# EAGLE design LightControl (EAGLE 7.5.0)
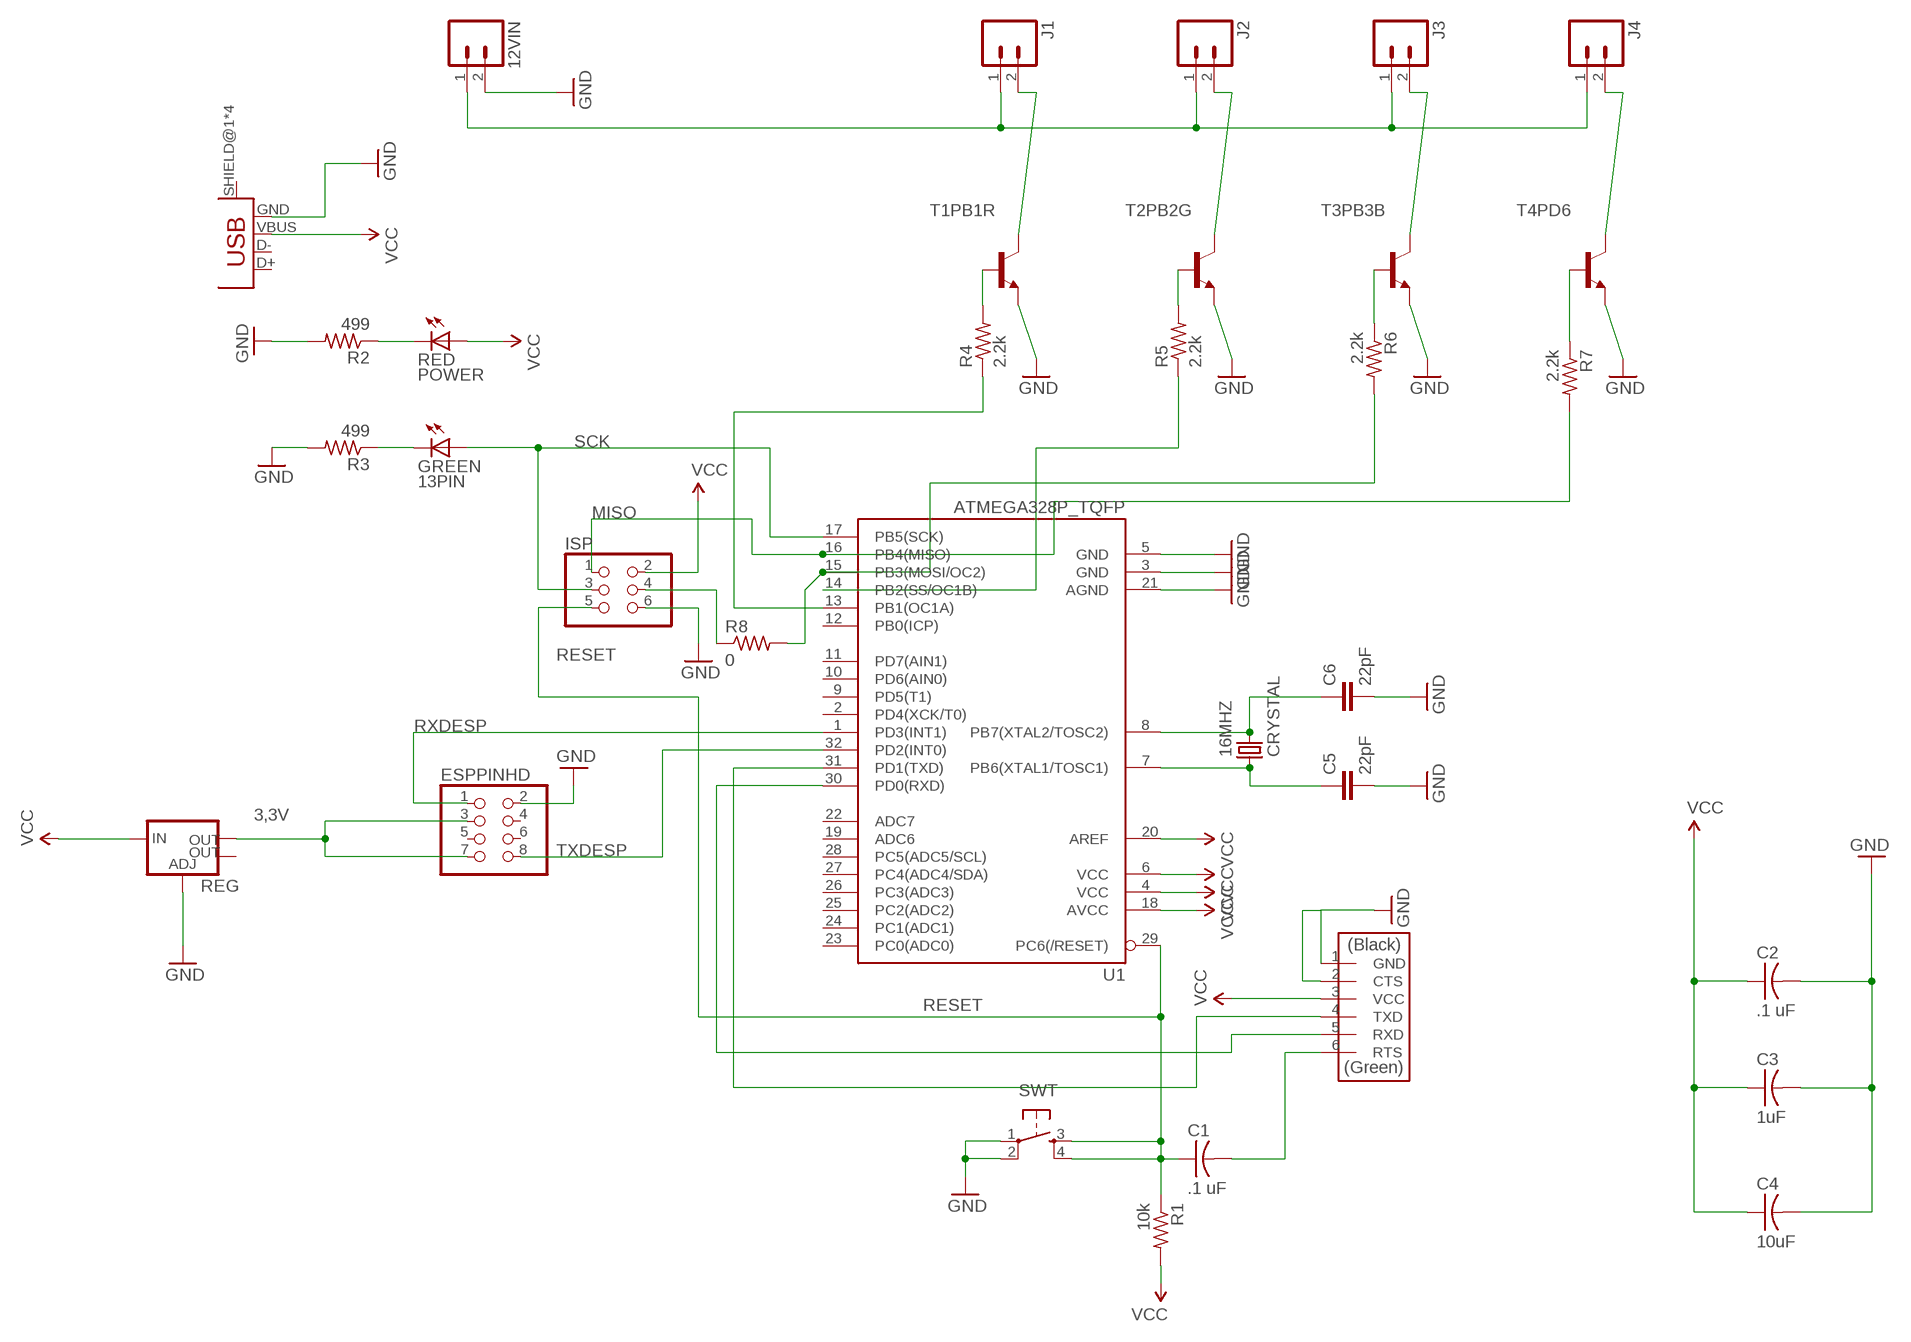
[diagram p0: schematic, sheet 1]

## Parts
12VIN  M025MM  [SCREWTERMINAL-5MM-2]
16MHZ  CRYSTAL  [2-SMD-5X3MM]
C1  .1 uF  CAP-US1206  [C1206]
C2  .1 uF  CAP-US1206  [C1206]
C3  1uF  CAP-US1206  [C1206]
C4  10uF  CAP-US1206  [C1206]
C5  22pF  CAPPTH1  [CAP-PTH-5MM]
C6  22pF  CAPPTH1  [CAP-PTH-5MM]
ESPPINHD  PINHD-2X4SMT  [2X04_SMT]
GREEN  13PIN  LEDFAB1206  [LED1206FAB]
ISP  PINHD-2X3-SMD  [2X03SMD]
J1  M025MM  [SCREWTERMINAL-5MM-2]
J2  M025MM  [SCREWTERMINAL-5MM-2]
J3  M025MM  [SCREWTERMINAL-5MM-2]
J4  M025MM  [SCREWTERMINAL-5MM-2]
R1  10k  RES-US1206FAB  [R1206FAB]
R2  499  RES-US1206FAB  [R1206FAB]
R3  499  RES-US1206FAB  [R1206FAB]
R4  2.2k  RES-US1206FAB  [R1206FAB]
R5  2.2k  RES-US1206FAB  [R1206FAB]
R6  2.2k  RES-US1206FAB  [R1206FAB]
R7  2.2k  RES-US1206FAB  [R1206FAB]
R8  0  RES-US1206FAB  [R1206FAB]
RED  POWER  LEDFAB1206  [LED1206FAB]
REG  V_REG_LM1117SOT223  [SOT223]
SWT  6MM_SWITCH6MM_SWITCH  [6MM_SWITCH]
T1PB1R  -NPN-TO220V  [TO220V]
T2PB2G  -NPN-TO220V  [TO220V]
T3PB3B  -NPN-TO220V  [TO220V]
T4PD6  -NPN-TO220V  [TO220V]
U1  ATMEGA328P_TQFP  [TQFP32-08]
U$1  FTDI-SMD-HEADER  [1X06SMD]
U$2  USB_MINIB  [USB_MINIB]

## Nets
3,3V: ESPPINHD.3 ESPPINHD.7 REG.2(OUT)
GND: 12VIN.2 C2.2 C3.2 C4.2 C5.2 C6.2 ESPPINHD.2 ISP.6 R2.2 R3.2 REG.1(ADJ) SWT.1(P) SWT.2(P1) T1PB1R.3(E) T2PB2G.3(E) T3PB3B.3(E) T4PD6.3(E) U1.3(GND) U1.5(GND) U1.21(AGND) U$1.1(GND) U$1.2(CTS) U$2.GND
MISO: ISP.1 R7.2 U1.16(PB4(MISO))
MOSI: R6.2 R8.2 U1.15(PB3(MOSI/OC2))
N$1: U1.30(PD0(RXD)) U$1.5(RXD)
N$2: 16MHZ.P$2 C6.1 U1.8(PB7(XTAL2/TOSC2))
N$3: 16MHZ.P$1 C5.1 U1.7(PB6(XTAL1/TOSC1))
N$4: C1.2 U$1.6(RTS)
N$5: R2.1 RED.2(C)
N$6: U1.31(PD1(TXD)) U$1.4(TXD)
N$7: ISP.4 R8.1
N$8: GREEN.2(C) R3.1
N$9: R4.2 T1PB1R.1(B)
N$10: R5.2 T2PB2G.1(B)
N$11: R6.1 T3PB3B.1(B)
N$12: R7.1 T4PD6.1(B)
N$13: R4.1 U1.13(PB1(OC1A))
N$14: R5.1 U1.14(PB2(SS/OC1B))
N$15: J1.2 T1PB1R.2(C)
N$16: J2.2 T2PB2G.2(C)
N$17: J3.2 T3PB3B.2(C)
N$18: J4.2 T4PD6.2(C)
N$19: 12VIN.1 J1.1 J2.1 J3.1 J4.1
RESET: C1.1 ISP.5 R1.1 SWT.3(S) SWT.4(S1) U1.29(PC6(/RESET))
RXDESP: ESPPINHD.1 U1.1(PD3(INT1))
SCK: GREEN.1(A) ISP.3 U1.17(PB5(SCK))
TXDESP: ESPPINHD.8 U1.32(PD2(INT0))
VCC: C2.1 C3.1 C4.1 ISP.2 R1.2 RED.1(A) REG.3(IN) U1.4(VCC) U1.6(VCC) U1.18(AVCC) U1.20(AREF) U$1.3(VCC) U$2.VBUS
Unconnected: ESPPINHD.4 ESPPINHD.5 ESPPINHD.6 REG.4(OUT) U1.2(PD4(XCK/T0)) U1.9(PD5(T1)) U1.10(PD6(AIN0)) U1.11(PD7(AIN1)) U1.12(PB0(ICP)) U1.19(ADC6) U1.22(ADC7) U1.23(PC0(ADC0)) U1.24(PC1(ADC1)) U1.25(PC2(ADC2)) U1.26(PC3(ADC3)) U1.27(PC4(ADC4/SDA)) U1.28(PC5(ADC5/SCL)) U$2.D+ U$2.D- U$2.SHIELD@1(SHIELD) U$2.SHIELD@2(SHIELD) U$2.SHIELD@3(SHIELD) U$2.SHIELD@4(SHIELD)

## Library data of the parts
12VIN J1-J4 = SparkFun-Connectors:M02: Standard 2-pin 0.1" header. Use with; STOREFRONT_ID: PRT-08432
16MHZ = fab:CRYSTAL
C1-C4 = fab:CAP-US
C5 C6 = SparkFun-Capacitors:CAP: Capacitor
ESPPINHD = pinhead+:PINHD-2X4: PIN HEADER
GREEN RED = fab:LED: LED
ISP = fab:PINHD-2X3-SMD: PIN HEADER
R1-R8 = fab:RES-US: Resistor (US Symbol)
REG = SparkFun-PowerIC:V_REG_LM1117: Voltage Regulator LM1117 Standard adjustable voltage regulator but in SMD form. Spark Fun Electronics SKU : COM-00595; PROD_ID: VREG-08170
SWT = fab:6MM_SWITCH: OMRON SWITCH
T1PB1R T2PB2G T3PB3B T4PD6 = transistor:*-NPN-: NPN Transistror BF959 corrected 2008.03.06
U1 = SparkFun-DigitalIC:ATMEGA328P_TQFP; PROD_ID: IC-09069
U$1 = fab:FTDI-SMD-HEADER
U$2 = fab:USB_MINIB

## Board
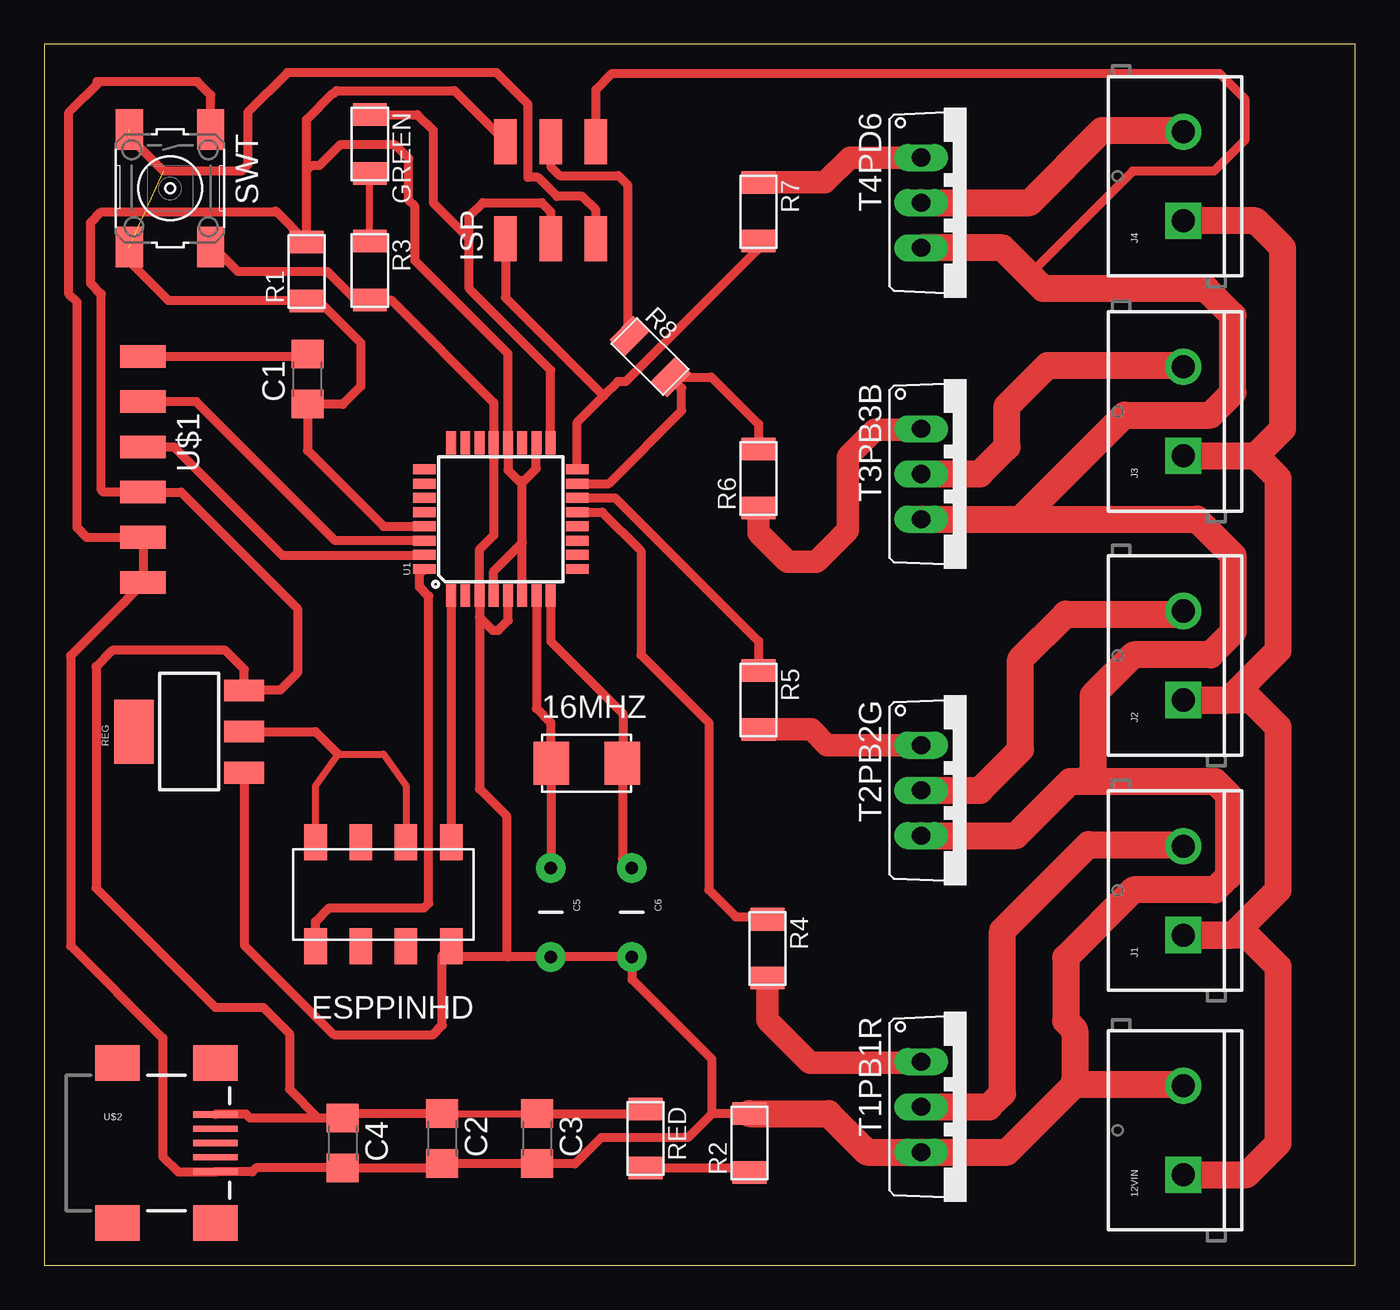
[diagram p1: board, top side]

Size 73.66 x 68.58 mm. Coordinates in mm from the lower left corner, seen from the top.
Outline: 0,0 73.66,0 73.66,68.58 0,68.58 0,0
Copper layers (1*16): Top 0.035mm / dielectric 1.5mm / Bottom 0.035mm
Design rules "default": minimum track width 10mil, minimum drill 24mil, track to track 8mil, track to pad 8mil, pad to pad 8mil, via to via 8mil, smd to smd 8mil, copper to edge 40mil, drill to drill 8mil, minimum pad ring 10mil, minimum via ring 8mil, stop-mask expansion 4mil, vias tented up to drill 0mil, thermal gap 10mil

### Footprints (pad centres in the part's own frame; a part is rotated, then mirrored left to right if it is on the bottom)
SCREWTERMINAL-5MM-2 = drill 1.3 pad 2.032 square: 1 0,0 | drill 1.3 pad 2.032: 2 5,0
2-SMD-5X3MM = smd 2 x 2.4: P$1 -2,0; P$2 2,0
C1206 = smd 1.6 x 1.8: 1 -1.4,0; 2 1.4,0
CAP-PTH-5MM = drill 0.7 pad 1.651: 1 -2.5,0; 2 2.5,0
2X04_SMT = smd 1.27 x 2.032: 1 -3.81,-2.921; 2 -3.81,2.921; 3 -1.27,-2.921; 4 -1.27,2.921; 5 1.27,-2.921; 6 1.27,2.921; 7 3.81,-2.921; 8 3.81,2.921
LED1206FAB = smd 1.27 x 1.905: 1 -1.651,0; 2 1.651,0
2X03SMD = smd 2.54 x 1.27: 1 -2.54,2.54; 2 2.92,2.54; 3 -2.54,0; 4 2.92,0; 5 -2.54,-2.54; 6 2.92,-2.54
R1206FAB = smd 1.27 x 1.905: 1 -1.651,0; 2 1.651,0
SOT223 = smd 1.219 x 2.235: 1 -2.311,-3.099; 2 0,-3.099; 3 2.311,-3.099 | smd 3.6 x 2.2: 4 0,3.099
6MM_SWITCH = smd 2.286 x 1.524: 1 -3.302,2.286; 2 3.302,2.286; 3 -3.302,-2.286; 4 3.302,-2.286
TO220V = drill 1.016 long: 1 -2.54,-2.54; 2 0,-2.54; 3 2.54,-2.54
TQFP32-08 = smd 1.27 x 0.559: 1 -4.293,2.8; 2 -4.293,2; 3 -4.293,1.2; 4 -4.293,0.4; 5 -4.293,-0.4; 6 -4.293,-1.2; 7 -4.293,-2; 8 -4.293,-2.8; 17 4.293,-2.8; 18 4.293,-2; 19 4.293,-1.2; 20 4.293,-0.4; 21 4.293,0.4; 22 4.293,1.2; 23 4.293,2; 24 4.293,2.8 | smd 0.559 x 1.27: 9 -2.8,-4.293; 10 -2,-4.293; 11 -1.2,-4.293; 12 -0.4,-4.293; 13 0.4,-4.293; 14 1.2,-4.293; 15 2,-4.293; 16 2.8,-4.293; 25 2.8,4.293; 26 2,4.293; 27 1.2,4.293; 28 0.4,4.293; 29 -0.4,4.293; 30 -1.2,4.293; 31 -2,4.293; 32 -2.8,4.293
1X06SMD = smd 2.54 x 1.27: 1 0,6.35; 2 0,3.81; 3 0,1.27; 4 0,-1.27; 5 0,-3.81; 6 0,-6.35
USB_MINIB = smd 2.5 x 0.35: D+ 3.77,0; D- 3.77,0.8; GND 3.77,-1.6; ID 3.77,-0.8; VBUS 3.77,1.6 | smd 2.5 x 2: SHIELD@1 -1.73,-4.5; SHIELD@2 -1.73,4.5; SHIELD@3 3.77,4.5; SHIELD@4 3.77,-4.5

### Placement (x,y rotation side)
12VIN  64.01,5.08 90 top
16MHZ  30.48,28.19 0 top
C1  14.78,49.78 90 top
C2  22.35,7.11 270 top
C3  27.69,7.11 270 top
C4  16.76,6.86 270 top
C5  28.45,19.81 270 top
C6  33.02,19.81 270 top
ESPPINHD  19.05,20.83 180 top
GREEN  18.29,62.99 270 top
ISP  28.45,60.2 90 top
J1  64.01,18.54 90 top
J2  64.01,31.75 90 top
J3  64.01,45.47 90 top
J4  64.01,58.67 90 top
R1  14.73,55.83 90 top
R2  39.62,6.86 90 top
R3  18.29,55.88 270 top
R4  40.64,17.78 270 top
R5  40.13,31.75 270 top
R6  40.13,44.2 90 top
R7  40.13,59.18 270 top
R8  34.04,51.05 315 top
RED  33.78,7.11 270 top
REG  8.13,29.97 90 top
SWT  7.06,60.5 270 top
T1PB1R  51.82,8.89 270 top
T2PB2G  51.82,26.67 270 top
T3PB3B  51.82,44.45 270 top
T4PD6  51.82,59.69 270 top
U1  25.65,41.91 90 top
U$1  5.54,44.7 180 top
U$2  5.84,6.86 0 top

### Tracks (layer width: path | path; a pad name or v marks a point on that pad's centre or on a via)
3,3V
  Top 0.406: ESPPINHD.7 15.24,26.92 16.51,28.7 19.05,28.7 20.32,26.92 ESPPINHD.3
  Top 0.508: REG.2 15.24,29.97 16.51,28.7
GND
  Top 0.508: 26.06,17.31 C5.2 C6.2 33.02,16.05 37.49,11.58 37.49,8.53 37.52,8.51 | 26.06,17.31 23.45,17.31 ESPPINHD.2 22.35,17.4 22.35,13.46 21.84,12.95 16.26,12.95 11.23,17.98 REG.1 | U1.3 24.45,26.75 25.96,25.25 25.96,17.41 26.06,17.31 | U1.3 24.45,36.4 25.2,35.66 25.5,35.66 26.06,36.22 U1.5 | U1.21 25.25,45.67 | 25.25,45.67 25.25,41 24.43,40.18 24.43,37.64 U1.3 | R2.2 37.52,8.51 | 37.52,8.51 36.17,7.16 31.29,7.16 29.82,5.69 27.71,5.69 C3.2 C2.2 22.1,5.46 C4.2 11.91,5.46 11.68,5.23 9.64,5.23 U$2.GND 9.59,5.23 7.52,5.23 6.66,6.1 6.66,12.75 1.47,17.93 1.47,34.24 4.32,37.08 U$1.1 U$1.2 2.39,40.89 1.83,41.45 1.83,54.1 1.37,54.56 1.37,64.77 3.1,66.5 | 25.25,45.67 25.25,45.68 25.25,48.46 19.48,54.23 R3.2 17.5,54.23 15.9,55.83 10.87,55.83 9.5,57.2 SWT.2 | SWT.1 9.35,65.73 8.59,66.5 3.1,66.5 | 3.1,66.5 2.95,66.5 | ISP.6 30.99,66.04 31.9,66.95 66.04,66.95 67.46,65.53 67.46,63.2 65.73,61.47 61.16,61.47 55.35,55.65
  Top 1.524: 58.17,10.16 57.91,10.16 54.1,6.35 T1PB1R.3 46.23,6.35 44.07,8.51 R2.2 | 58.17,10.16 63.93,10.16 12VIN.2 | T2PB2G.3 54.61,24.13 57.66,27.18 58.42,27.18 | 58.42,27.18 65.79,27.18 66.55,26.42 66.55,21.84 65.79,21.08 61.21,21.08 57.4,17.27 57.4,13.72 57.91,13.21 57.91,10.41 58.17,10.16 | 58.42,27.18 58.93,27.69 58.93,32 61.21,34.29 65.53,34.29 66.8,35.56 66.8,39.88 64.77,41.91 T3PB3B.3 54.86,41.91 60.71,47.75 65.53,47.75 66.8,49.02 66.8,53.34 65.28,54.86 56.13,54.86 55.35,55.65 53.85,57.15 T4PD6.3
MISO
  Top 0.508: U1.16 29.95,47.35 31.43,48.83 | ISP.1 25.91,54.36 31.43,48.83 | R7.2 40.13,57.1 32.66,49.63 32.23,49.63 31.43,48.83
MOSI
  Top 0.508: U1.15 31.72,43.91 35.81,48.01 35.81,49.28 R8.2 37.49,49.89 40.13,47.24 R6.2
N$1
  Top 0.508: U1.30 16.34,40.71 8.53,48.51 U$1.5
N$2
  Top 0.508: U1.8 28.45,35.05 32.51,30.99 32.51,28.23 16MHZ.P$2 32.48,22.85 C6.1
N$3
  Top 0.508: U1.7 27.65,31.27 28.45,30.48 28.45,28.23 16MHZ.P$1 28.48,22.34 C5.1
N$4
  Top 0.508: U$1.6 14.65,51.05 C1.2
N$5
  Top 0.508: RED.2 40.26,5.46 40.39,5.33 39.75,5.33 R2.1
N$6
  Top 0.508: U$1.4 7.26,45.97 13.36,39.88 21.33,39.88 U1.31
N$7
  Top 0.508: ISP.4 28.45,61.72 28.96,61.21 32.26,61.21 32.77,60.71 32.77,52.32 R8.1
N$8
  Top 0.406: R3.1 GREEN.2
N$9
  Top 1.27: R4.2 40.64,13.77 43.03,11.38 49.23,11.38 T1PB1R.1
N$10
  Top 1.27: R5.2 43.1,30.1 43.99,29.21 T2PB2G.1
N$11
  Top 1.27: R6.1 40.13,41.15 41.76,39.52 43.38,39.52 45.16,41.3 45.16,45.41 46.69,46.94 49.23,46.94 T3PB3B.1
N$12
  Top 1.27: R7.1 43.87,60.83 45.26,62.23 T4PD6.1
N$13
  Top 0.508: U1.13 31.35,42.31 33.53,40.13 33.53,34.29 37.34,30.48 37.34,21.08 38.86,19.56 40.51,19.56 R4.1
N$14
  Top 0.508: U1.14 32.07,43.11 40.13,35.05 R5.1
N$15
  Top 1.524: T1PB1R.2 53.09,8.89 53.85,9.65 53.85,18.8 58.67,23.62 63.93,23.62 J1.2
N$16
  Top 1.524: T2PB2G.2 52.58,26.67 54.86,28.96 54.86,34.04 57.4,36.58 63.83,36.58 J2.2
N$17
  Top 1.524: T3PB3B.2 52.58,44.45 54.1,45.97 54.1,48.26 56.39,50.55 63.93,50.55 J3.2
N$18
  Top 1.524: T4PD6.2 55.37,59.69 59.44,63.75 63.93,63.75 J4.2
N$19
  Top 1.524: 12VIN.1 67.56,5.08 69.34,6.86 69.34,16.76 67.56,18.54 J1.1 66.8,18.54 69.34,21.08 69.34,30.23 67.82,31.75 J2.1 66.55,31.75 69.34,34.54 69.34,44.2 68.07,45.47 | J3.1 68.07,45.47 | 68.07,45.47 69.6,46.99 69.6,57.15 68.07,58.67 J4.1
RESET  (2 unrouted)
  Top 0.508: U1.29 19.05,41.5 14.78,45.77 C1.1 14.8,48.36 16.76,48.36 17.78,49.38 17.78,51.82 15.42,54.18 R1.1 14.71,54.2 6.96,54.2 4.78,56.39 SWT.4 | ISP.5 30.99,59.28 30.23,60.05 28.8,60.05 27.74,61.11 27.18,61.11 27.18,65.23 25.4,67 13.66,67 11.43,64.77 11.43,61.82 11.07,61.47 6.71,61.47 4.78,63.4
RXDESP
  Top 0.508: U1.1 ESPPINHD.1
SCK
  Top 0.508: U1.17 28.45,50.29 23.88,54.86 23.88,57.66 | 23.88,57.66 23.88,58.93 24.64,59.69 27.94,59.69 28.45,59.18 ISP.3 | GREEN.1 20.95,64.64 21.84,63.75 21.84,59.69 23.88,57.66
TXDESP
  Top 0.508: ESPPINHD.8 15.24,19.3 16,20.07 21.34,20.07 21.59,20.32 21.59,37.59 21.08,38.1 21.08,38.83 U1.32
VCC
  Top 0.406: C2.1 C3.1
  Top 0.508: C3.1 33.53,8.51 RED.1 | C2.1 17.02,8.51 C4.1 15.39,8.26 | 15.39,8.26 11.55,8.26 11.33,8.48 9.64,8.48 U$2.VBUS | 15.39,8.26 13.77,9.88 13.77,13.01 12.29,14.48 9.6,14.48 2.9,21.18 2.9,33.63 3.81,34.54 10.16,34.54 11.23,33.48 REG.3 11.25,32.31 13.26,32.31 14.22,33.27 14.22,36.88 7.67,43.43 U$1.3 3.3,43.43 3.2,43.54 3.2,54.56 2.59,55.17 2.59,58.57 3.2,59.18 12.93,59.18 12.98,59.23 R1.2 14.73,61.52 | 14.73,61.52 14.73,64.36 16.2,65.84 16.26,65.84 16.41,65.99 23.04,65.99 ISP.2 | 14.73,61.52 14.99,61.77 15.44,61.77 16.61,62.94 19.71,62.94 20.47,62.18 20.47,59.84 20.83,59.49 20.83,56.44 26.05,51.21 U1.20 26.05,44.66 26.62,44.09 26.98,44.09 | 26.98,44.09 27.64,44.76 27.64,46.18 U1.18 | U1.6 26.85,40.59 | 26.85,40.59 26.85,43.97 26.98,44.09 | U1.4 25.25,38.99 26.85,40.59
